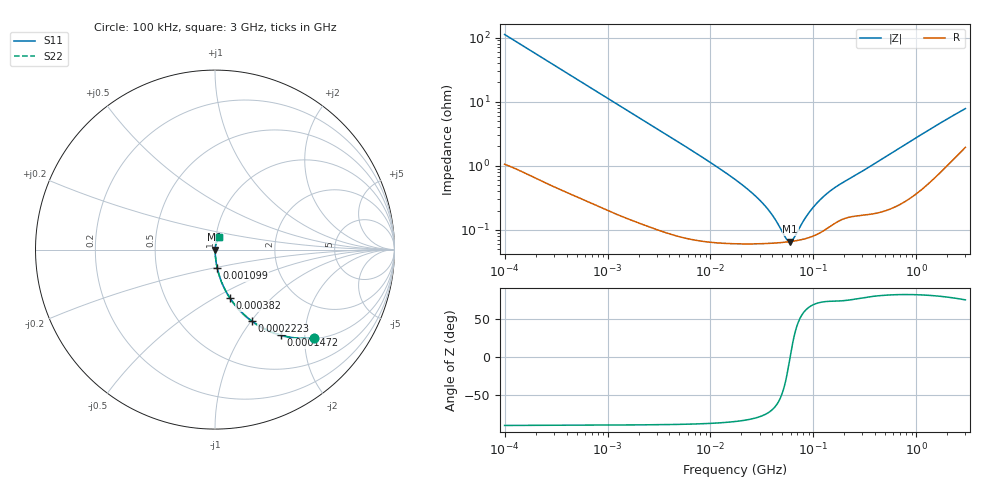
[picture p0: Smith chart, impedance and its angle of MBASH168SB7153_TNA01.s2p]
! MBASH168SB7153_TNA01  S-PARAMETER MODEL  ( Standard Model )
! Model Generated by TAIYO YUDEN Corporation (http://www.ty-top.com)
! Version 1.0
! TAIYO YUDEN Control No. 220601
! Copyright(c) 2013 TAIYO YUDEN CO.,LTD. All Rights Reserved.
! Product Description (link to TY-COMPAS)
! https://ds.yuden.co.jp/TYCOMPAS/or/detail?pn=MBASH168SB7153KTNA01&u=M
! Products Name : Multilayer Ceramic Capacitors
! Characteristics :
!  Capacitance : 0.015 [uF] , Rated Voltage : 100 [V] , TCC : X7R
!  Case Size : 1.6 x 0.8 / 0.063 x 0.031 [mm/inch] , Thickness : 0.8 / 0.031 [mm/inch]
!  (Conditions: Temperature = 25 [degC] , DC Bias Voltage = 0 [V])
! External Node Assignments :
!  1  o---| |---o  2
! GND o---------o GND
! Frequency Range : 100kHz  -  3GHz  [ 401 STEP ]
# MHZ S RI R 50
! Freq[MHz].  S11 Real  S11 Imag  S21 Real  S21 Imag  S12 Real  S12 Imag  S22 Real  S22 Imag
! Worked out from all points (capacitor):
!   401 points, 100 kHz to 3 GHz, reference 50 ohm
!   read as one part in series: C = 14.2 nF near 105.3 kHz
!   lowest |Z| = 65.8 mohm at 59.68 MHz (marker M1)
!   series resonance near 59.4 MHz, so ESL is about 500 pH
!   S11 on the Smith chart (normalised r, x): 100 kHz: 1.02, -2.23; 147.2 kHz: 1.02, -1.52; 222.3 kHz: 1.01, -1.01; 382 kHz: 1.01, -0.59; 1.099 MHz: 1.00, -0.21; 3 GHz: 1.04, +0.15
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0.1  0.5541 -0.4923  0.4459 0.4923  0.4459 0.4923  0.5541 -0.4923
0.147195  0.3676 -0.4768  0.6324 0.4768  0.6324 0.4768  0.3676 -0.4768
0.222319  0.2058 -0.3985  0.7942 0.3985  0.7942 0.3985  0.2058 -0.3985
0.381967  0.0831 -0.2693  0.9169 0.2693  0.9169 0.2693  0.0831 -0.2693
0.562235  0.0415 -0.192  0.9585 0.192  0.9585 0.192  0.0415 -0.192
1.09883  0.0124 -0.1019  0.9876 0.1019  0.9876 0.1019  0.0124 -0.1019
3.161081  0.00229 -0.0361  0.9977 0.0361  0.9977 0.0361  0.00229 -0.0361
17.7727  0.000642 -0.00591  0.9994 0.00591  0.9994 0.00591  0.000642 -0.00591
25.49486  0.000618 -0.00369  0.9994 0.00369  0.9994 0.00369  0.000618 -0.00369
32.98988  0.000617 -0.00242  0.9994 0.00242  0.9994 0.00242  0.000617 -0.00242
41.60216  0.000624 -0.00141  0.9994 0.00141  0.9994 0.00141  0.000624 -0.00141
53.83243  0.000645 -0.000383  0.9994 0.000383  0.9994 0.000383  0.000645 -0.000383
56.67997  0.000651 -0.000182  0.9993 0.000182  0.9993 0.000182  0.000651 -0.000182
59.67813  0.000657 1.83e-05  0.9993 -1.83e-05  0.9993 -1.83e-05  0.000657 1.83e-05
64.47533  0.000669 0.000319  0.9993 -0.000319  0.9993 -0.000319  0.000669 0.000319
81.30716  0.000722 0.00124  0.9993 -0.00124  0.9993 -0.00124  0.000722 0.00124
97.38194  0.000793 0.002  0.9992 -0.002  0.9992 -0.002  0.000793 0.002
122.8043  0.000957 0.00306  0.999 -0.00306  0.999 -0.00306  0.000957 0.00306
158.9065  0.00126 0.0043  0.9987 -0.0043  0.9987 -0.0043  0.00126 0.0043
547.5153  0.00231 0.0148  0.9977 -0.0148  0.9977 -0.0148  0.00231 0.0148
1658.39  0.00933 0.0436  0.9907 -0.0436  0.9907 -0.0436  0.00933 0.0436
3000  0.0244 0.0722  0.9756 -0.0722  0.9756 -0.0722  0.0244 0.0722
